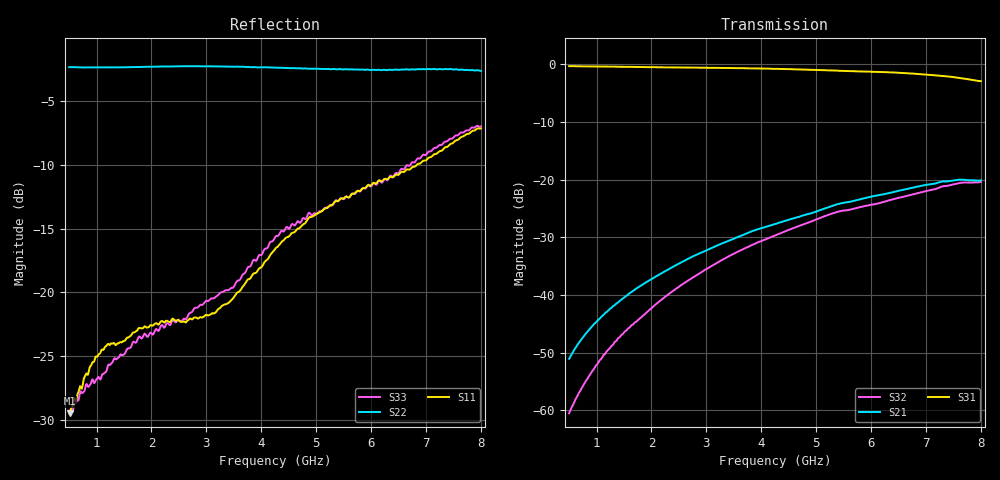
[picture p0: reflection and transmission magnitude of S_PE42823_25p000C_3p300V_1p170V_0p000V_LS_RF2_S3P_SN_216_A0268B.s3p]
! Device ID: PE42823
! File Path: z:\PE42823\DSPLOTS2\25p000C\3p300\LS_RF2\PE42823_25p000C_3p300V_1p170V_0p000V_LS_RF2_S3P_SN_216_A0268B.s3p
! Serial: 216
! Lot: A0268B
! Temp: 25.000C
! VDD: 3.300
! VSS: 0.000
! Control_Hi: 1.170
! Control_Lo: 0.000
! Logic State: LS_RF2
! Port 1: RFC
! Port 2: RF1
! Port 3: RF2
! ThroughPath:1-3
! IDD: 0.000123774953
! ISS/IDD2: -2.46129219e-009
! IDMM3/IDD3: 0
! Comment:
#  Hz  S  RI  R  50
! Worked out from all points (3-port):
!   751 points, 500 MHz to 8 GHz, reference 50 ohm
!   strongest paths, dB at 500 MHz, 2.37 GHz, 4.25 GHz, 6.13 GHz, 8 GHz:
!     S31: -0.4, -0.6, -0.8, -1.4, -2.9
!     S21: -51.1, -35.2, -27.7, -22.7, -20.1
!     S32: -60.5, -39.5, -29.7, -24.1, -20.4
!   lowest |S11| = -29.5 dB at 510 MHz (marker M1), VSWR 1.07, Z = 52.5 - j2.37 ohm
!   |S11| at or under -10 dB: start of sweep to 6.834 GHz
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5e8  0.0252 -0.0228  -0.00017 0.00277  0.9482 -0.1449
     -0.000184 0.00279  -0.7522 0.127  -0.00033 0.000891
     0.949 -0.1449  -0.000331 0.000882  0.0239 -0.0236
5.1e8  0.0248 -0.0226  -0.000194 0.00284  0.948 -0.1473
       -0.000185 0.00284  -0.7524 0.1293  -0.000352 0.000902
       0.9484 -0.1478  -0.000341 0.000908  0.0245 -0.0237
1.15e9  0.0198 -0.0576  -0.000565 0.00687  0.8969 -0.3215
        -0.000562 0.00688  -0.7106 0.2726  -0.00149 0.00269
        0.8965 -0.3223  -0.00146 0.00268  0.00346 -0.0483
2.08e9  -0.0144 -0.0742  -0.00058 0.0144  0.7678 -0.5437
        -0.000586 0.0144  -0.6065 0.4694  -0.00375 0.00744
        0.7666 -0.5437  -0.00371 0.00741  -0.0466 -0.0545
3.15e9  -0.0601 -0.057  0.00208 0.026  0.5559 -0.7434
        0.00208 0.0261  -0.4219 0.643  -0.00437 0.0179
        0.5558 -0.7438  -0.00434 0.0179  -0.0794 -0.0523
4.25e9  -0.1465 -0.0173  0.0117 0.0393  0.2766 -0.8666
        0.0117 0.0394  -0.2063 0.7314  0.00306 0.0326
        0.2749 -0.8681  0.00317 0.0326  -0.1414 -0.0837
4.99e9  -0.2 0.0277  0.0213 0.0477  0.072 -0.8861
        0.0214 0.0479  -0.0584 0.7506  0.0143 0.0427
        0.0712 -0.8868  0.0144 0.0425  -0.1933 -0.064
6.1e9  -0.2506 0.0958  0.0468 0.055  -0.2231 -0.8272
       0.047 0.0553  0.1895 0.7191  0.041 0.0462
       -0.223 -0.8282  0.0411 0.046  -0.2546 0.0705
7.3e9  -0.2315 0.2765  0.082 0.0492  -0.4865 -0.6221
       0.0824 0.0496  0.4431 0.6028  0.0786 0.0384
       -0.4876 -0.6225  0.0785 0.0379  -0.2738 0.2643
8e9  -0.139 0.4163  0.0925 0.0331  -0.5442 -0.4613
     0.0926 0.0332  0.5298 0.5136  0.0939 0.017
     -0.5444 -0.4593  0.0938 0.0167  -0.2404 0.377
